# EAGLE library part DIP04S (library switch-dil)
DIL/CODE SWITCH
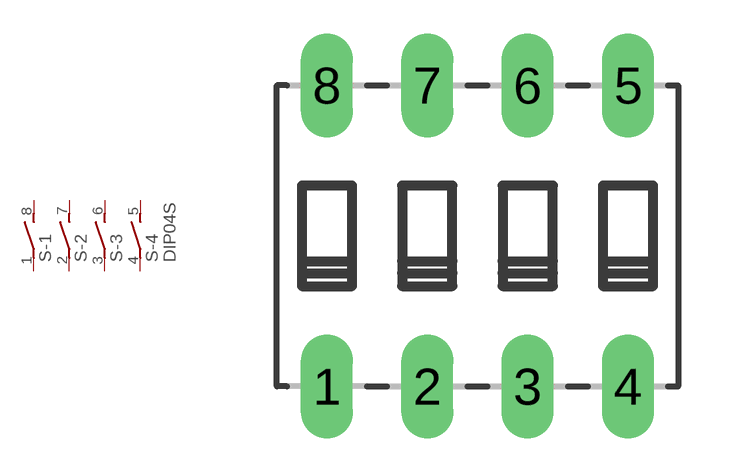
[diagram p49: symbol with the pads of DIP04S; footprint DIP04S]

Designator prefix S; gates -1=S -2=S -3=S -4=S+V

## DIP04S (OC_FARNELL: unknown; OC_NEWARK: unknown)  [DIP04S]
1  -1:1  pas
2  -2:1  pas
3  -3:1  pas
4  -4:1  pas
5  -4:2  pas
6  -3:2  pas
7  -2:2  pas
8  -1:2  pas

## Footprint DIP04S (pad centres in mm)
DIL/CODE SWITCH small
drill 0.813 long: 1 -3.81,-3.81; 2 -1.27,-3.81; 3 1.27,-3.81; 4 3.81,-3.81; 5 3.81,3.81; 6 1.27,3.81; 7 -1.27,3.81; 8 -3.81,3.81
